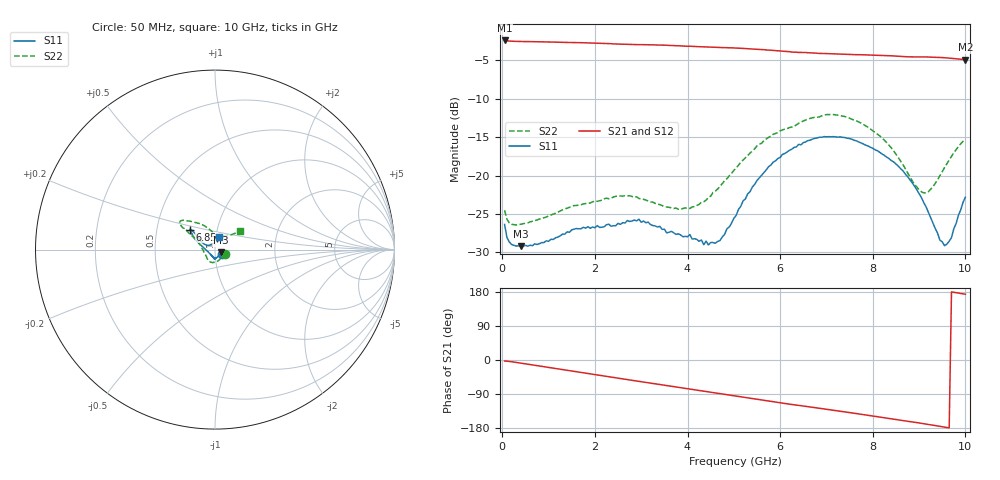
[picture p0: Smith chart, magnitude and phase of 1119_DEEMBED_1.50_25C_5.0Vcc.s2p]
!Hittite Microwave Corp.
!Digital Attenuator/PhaseShifter Rev 1.4.0
!Filename: C:\DATA\DATA\1119_DEEMBED_1.50_25C_5.0Vcc.s2p
!VNA ID: Agilent Technologies,N5224A,MY51441122,A.10.45.03
!Device type:
!2 Port Calibration.
!Temp(C): 25
!Lot Number:
!Serial Number:
!Operator:
!Misc:
!Attenuator:  1.500
# GHZ S DB R 50.0
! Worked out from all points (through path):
!   200 points, 50 MHz to 10 GHz, reference 50 ohm
!   highest |S21| = -2.40 dB at 50 MHz (marker M1); lowest = -4.9 dB at 10 GHz (marker M2)
!   group delay of S21, straight-line fit = 50.9 ps
!   lowest |S11| = -29.2 dB at 400 MHz (marker M3), VSWR 1.07, Z = 53.2 - j1.54 ohm
!   |S11| at or under -10 dB: start of sweep to end of sweep
!   |S22| runs from -26.4 to -12.1 dB; largest |S21 - S12| = 0.0018
!   S11 on the Smith chart (normalised r, x): 50 MHz: 1.09, -0.05; 6.85 GHz: 0.74, +0.17; 10 GHz: 1.03, +0.14
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0.05  -26.37 -29.8  -2.40 -2.6  -2.39 -2.6  -24.52 -21.8
0.15  -28.64 -21.3  -2.48 -3.7  -2.48 -3.7  -26.15 -17.3
0.4  -29.20 -24.7  -2.53 -8.2  -2.53 -8.2  -26.34 -23.1
1.75  -26.74 -79.7  -2.70 -34.0  -2.70 -34.0  -23.69 -75.8
2.75  -25.98 -91.2  -2.92 -52.7  -2.92 -52.8  -22.63 -111.1
3.4  -26.61 -100.8  -3.00 -64.8  -3.00 -64.8  -23.79 -134.5
3.55  -27.46 -102.4  -3.03 -67.7  -3.03 -67.7  -24.10 -138.7
4.05  -27.68 -110.8  -3.15 -76.9  -3.15 -77.0  -24.29 -162.3
4.45  -29.04 -133.2  -3.26 -84.4  -3.27 -84.4  -22.85 175.3
4.7  -28.47 -155.0  -3.32 -88.9  -3.33 -89.0  -21.43 162.9
5.05  -25.19 177.0  -3.39 -95.4  -3.41 -95.5  -19.00 152.9
5.75  -18.85 154.8  -3.65 -108.5  -3.67 -108.6  -15.03 147.2
6.7  -15.25 142.6  -4.02 -125.0  -4.03 -125.0  -12.47 143.8
6.85  -15.00 141.0  -4.09 -127.4  -4.10 -127.5  -12.35 143.3
7.65  -15.48 140.0  -4.25 -141.4  -4.26 -141.5  -12.89 134.8
8.35  -17.79 142.6  -4.39 -154.3  -4.39 -154.3  -16.03 117.5
8.75  -20.13 147.6  -4.53 -161.6  -4.53 -161.6  -19.60 101.0
9.1  -23.51 152.5  -4.55 -168.0  -4.56 -168.0  -22.26 79.1
9.3  -26.20 149.9  -4.58 -172.0  -4.59 -172.0  -21.43 62.4
9.55  -29.14 122.3  -4.65 -177.2  -4.66 -177.2  -18.96 45.4
9.7  -28.08 96.2  -4.73 179.7  -4.74 179.7  -17.50 40.4
10  -22.82 72.7  -4.90 173.5  -4.91 173.5  -15.27 37.1
